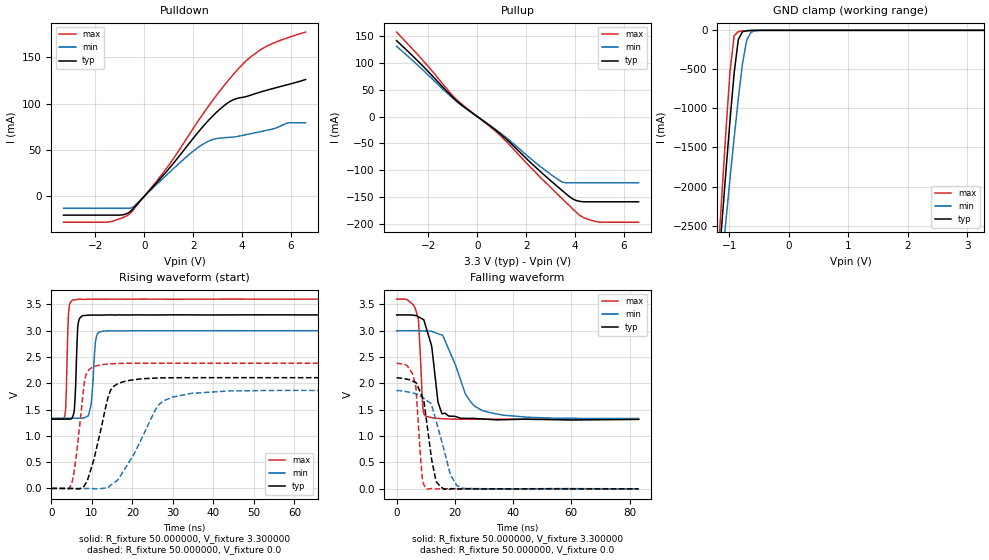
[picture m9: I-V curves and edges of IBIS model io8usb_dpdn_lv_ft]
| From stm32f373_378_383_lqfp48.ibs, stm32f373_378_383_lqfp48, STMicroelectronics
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|   Model io8usb_dpdn_lv_ft
[Model]  io8usb_dpdn_lv_ft
Model_type I/O
Polarity   Non-Inverting
Enable   Active-Low
Vinl =   0.990000V
Vinh =   2.310000V
Vmeas =  1.650000V
Cref =   50.000000pF
Rref =   100.000000M
Vref =   0.0V
C_comp   5.029800pF   4.851400pF   5.238000pF
[Temperature Range]   25.000000   0.125000k   -40.000000
[Pullup Reference]   3.300000V   3.000000V   3.600000V
[Pulldown Reference]   0.0V   0.0V   0.0V
[POWER Clamp Reference]   3.300000V   3.000000V   3.600000V
[GND Clamp Reference]   0.0V   0.0V   0.0V
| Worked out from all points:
|   slope of the pulldown table from 0 to 0.495 V, typ, clamps not added: 34.5 ohm
|   slope of the pullup table from 0 to 0.495 V, typ, clamps not added: 30.3 ohm
|   GND clamp passes 1 mA (typ) near -0.59 V on its own axis
|   rising waveform, R_fixture 50.000000, V_fixture 3.300000: 20-80 % time 564ps typ, 846ps min, 473ps max; typ from 1.32 V to 3.3 V
|   rising waveform, R_fixture 50.000000, V_fixture 0.0: 20-80 % time 3.84ns typ, 7.52ns min, 2.08ns max; typ from 0 V to 2.11 V
|   falling waveform, R_fixture 50.000000, V_fixture 3.300000: 20-80 % time 3.08ns typ, 7.43ns min, 1.2ns max; typ from 3.3 V to 1.32 V
|   falling waveform, R_fixture 50.000000, V_fixture 0.0: 20-80 % time 3.23ns typ, 5.44ns min, 1.75ns max; typ from 2.11 V to 0 V
[Pulldown]
|Voltage   I(typ)   I(min)   I(max)
-3.3V     -20.2mA    -12.85mA   -27.8mA
-1.5V     -20.2mA    -12.85mA   -27.7mA
-600mV    -16.97mA   -12.85mA   -19mA
-400mV    -11.64mA   -10.26mA   -12.92mA
900mV     26.39mA    22.6mA     29.76mA
2.1V      65.72mA    50.72mA    77.05mA
2.7V      83.87mA    60.28mA    99.79mA
3.3V      98.46mA    63.32mA    120.5mA
4.1V      107.1mA    66.16mA    144.4mA
4.8V      112.8mA    70.03mA    158.7mA
5.9V      120.7mA    79.32mA    171.3mA
6.6V      126mA      79.32mA    177.1mA
[Pullup]
|Voltage   I(typ)   I(min)   I(max)
-3.3V     140.6mA    130.2mA    156.5mA
-2.2V     92.45mA    85.22mA    102.9mA
-900mV    31.27mA    30.18mA    33.72mA
1V        -34.42mA   -32.42mA   -37.73mA
2.5V      -98.62mA   -89.74mA   -108.9mA
3.4V      -134.4mA   -119.6mA   -149.1mA
3.6V      -142.1mA   -122.8mA   -157.9mA
4V        -154.8mA   -122.8mA   -175.4mA
4.2V      -157.3mA   -122.8mA   -183.4mA
4.6V      -158.1mA   -122.8mA   -191.5mA
5V        -158.1mA   -122.8mA   -195.7mA
6.6V      -158.1mA   -122.8mA   -195.9mA
[GND_clamp]
|Voltage   I(typ)   I(min)   I(max)
-3.3V     -9.706A    -9.44A     -9.292A
-1.2V     -3.211A    -3.572A    -3.02A
-1.13V    -2.511A    -3.009A    -2.153A
-1.06V    -1.824A    -2.453A    -1.311A
-990mV    -1.16A     -1.907A    -534mA
-920mV    -548mA     -1.377A    -70.08mA
-850mV    -120.4mA   -876.3mA   -15.9mA
-780mV    -17.66mA   -431.2mA   -9.191mA
-710mV    -5.44mA    -131mA     -5.02mA
-640mV    -2.077mA   -25.74mA   -2.003mA
-570mV    -540.4uA   -6.318mA   -433.9uA
3.28V     0A         0A         0A
[POWER_clamp]
|Voltage   I(typ)   I(min)   I(max)
-3.28V    0A         0A         0A
0V        0A         0A         0A
[Ramp]
| variable   typ   min   max
dV/dt_r  1.26426/3.83200n   1.11846/7.51490n   1.42818/2.07729n
dV/dt_f  1.18482/3.07298n   0.99942/7.43357n   1.36710/1.17360n
R_load = 50.000000
[Rising Waveform]
R_fixture= 50.000000
V_fixture= 3.300000
V_fixture_min= 3.000000
V_fixture_max= 3.600000
|time   V(typ)   V(min)   V(max)
0s        1.318V     1.335V     1.321V
3.337ns   1.318V     1.335V     1.39V
4.171ns   1.318V     1.335V     3.255V
5.172ns   1.351V     1.335V     3.583V
5.839ns   1.708V     1.335V     3.588V
6.507ns   3.081V     1.334V     3.597V
7.674ns   3.285V     1.334V     3.597V
9.843ns   3.298V     1.614V     3.601V
11.85ns   3.297V     2.977V     3.6V
83.08ns   3.3V       3V         3.6V
[Rising Waveform]
R_fixture= 50.000000
V_fixture= 0.0
V_fixture_min= 0.0
V_fixture_max= 0.0
|time   V(typ)   V(min)   V(max)
0s        24.82nV    326.6nV    86.88nV
5.005ns   -2.526mV   3.56uV     84.51mV
6.173ns   -9.311mV   6.602uV    642.1mV
8.175ns   56.84mV    -637.3uV   2.037V
10.84ns   665.9mV    -8.136mV   2.325V
13.85ns   1.693V     16.32mV    2.366V
15.52ns   1.952V     110.4mV    2.373V
26.03ns   2.1V       1.539V     2.381V
29.86ns   2.105V     1.736V     2.381V
83.08ns   2.107V     1.864V     2.381V
[Falling Waveform]
R_fixture= 50.000000
V_fixture= 3.300000
V_fixture_min= 3.000000
V_fixture_max= 3.600000
|time   V(typ)   V(min)   V(max)
0s        3.3V       3V         3.6V
7.508ns   3.265V     3V         3.21V
9.009ns   3.219V     2.997V     1.574V
10.01ns   3.087V     2.995V     1.38V
12.01ns   2.718V     2.989V     1.351V
14.18ns   1.666V     2.946V     1.337V
15.68ns   1.422V     2.916V     1.331V
23.69ns   1.337V     1.793V     1.322V
29.36ns   1.326V     1.49V      1.321V
83.08ns   1.318V     1.335V     1.321V
[Falling Waveform]
R_fixture= 50.000000
V_fixture= 0.0
V_fixture_min= 0.0
V_fixture_max= 0.0
|time   V(typ)   V(min)   V(max)
0s        2.107V     1.864V     2.381V
3.67ns    2.08V      1.841V     2.337V
6.507ns   2.019V     1.806V     1.967V
8.842ns   1.745V     1.734V     199.4mV
10.51ns   1.201V     1.67V      -1.64mV
12.01ns   568.2mV    1.597V     7.191mV
13.68ns   131.2mV    1.265V     -3.059mV
18.52ns   -1.931mV   264.6mV    5.518mV
22.86ns   -764.7uV   9.867mV    905.6uV
83.08ns   24.82nV    326.6nV    86.88nV
